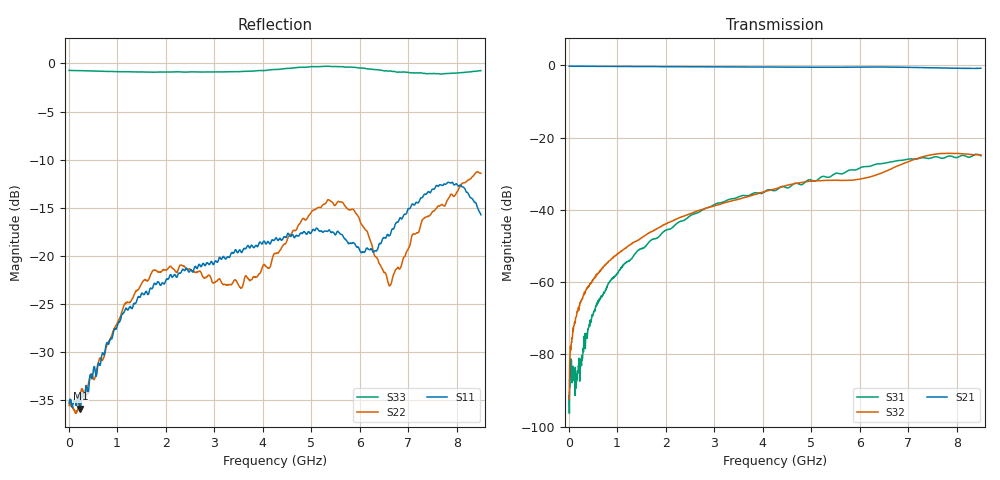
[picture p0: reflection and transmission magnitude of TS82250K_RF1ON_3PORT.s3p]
!Created with skrf (http://scikit-rf.org).
# GHz S RI R 50.0
!freq ReS11 ImS11 ReS12 ImS12 ReS13 ImS13
! ReS21 ImS21 ReS22 ImS22 ReS23 ImS23
! ReS31 ImS31 ReS32 ImS32 ReS33 ImS33
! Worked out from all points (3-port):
!   1601 points, 10 MHz to 8.5 GHz, reference 50 ohm
!   strongest paths, dB at 10 MHz, 2.132 GHz, 4.255 GHz, 6.378 GHz, 8.5 GHz:
!     S21: -0.2, -0.3, -0.4, -0.4, -0.8
!     S32: -92.4, -43.1, -34.2, -30.2, -24.7
!     S31: -91.5, -45.0, -34.6, -27.2, -25.0
!   lowest |S11| = -35.9 dB at 243.5 MHz (marker M1), VSWR 1.03, Z = 51.5 + j0.62 ohm
!   |S11| at or under -10 dB: start of sweep to end of sweep
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0.01  0.0172 -0.000587  0.9786 -0.0047  2.16e-05 3.25e-05
      0.9785 -0.00476  0.0166 0.00172  1.27e-05 5.26e-05
      1.5e-05 2.18e-05  1.21e-05 2.08e-05  -0.9197 0.00518
0.243475  0.0149 0.00601  0.9728 -0.069  -3.85e-05 6.52e-05
          0.9729 -0.069  0.018 0.00689  3.4e-05 0.00052
          -3.3e-05 6.45e-05  3.84e-05 0.000518  -0.9102 0.1129
0.6096063  0.0202 0.0184  0.9585 -0.1687  -0.000423 0.000312
           0.9585 -0.1686  0.0205 0.0187  -8.48e-05 0.00134
           -0.00048 0.000288  -8.95e-05 0.00134  -0.8707 0.2708
1.437381  0.0408 0.046  0.8882 -0.3828  -0.00235 0.0015
          0.8878 -0.3825  0.0406 0.0532  -0.000381 0.00384
          -0.00234 0.00149  -0.000397 0.00382  -0.6938 0.5779
3.034562  0.0919 0.0208  0.6324 -0.7172  -0.00679 0.0101
          0.6328 -0.7165  0.0504 0.0533  0.00266 0.0112
          -0.00677 0.0101  0.00277 0.0112  -0.1917 0.8826
4.255  0.1219 0.00724  0.3482 -0.8852  -0.00382 0.0181
       0.3479 -0.8847  0.0704 0.0754  0.0102 0.0167
       -0.0037 0.0182  0.0102 0.0167  0.2766 0.8865
5.602787  0.109 -0.0707  0.00603 -0.9458  0.000181 0.0317
          0.00608 -0.9457  0.1732 0.0797  0.022 0.0133
          0.000688 0.0317  0.022 0.0133  0.5265 0.8064
6.626894  -0.0509 -0.1174  -0.2788 -0.9094  0.0137 0.044
          -0.2793 -0.9087  0.0417 0.0563  0.0301 0.0205
          0.0145 0.0437  0.03 0.0204  0.6821 0.6078
7.831412  -0.1117 -0.2139  -0.5813 -0.7119  0.0408 0.0378
          -0.5812 -0.7128  0.1176 0.1604  0.0606 -0.00524
          0.0416 0.0368  0.0608 -0.00518  0.8538 0.2401
8.5  -0.0747 -0.1455  -0.7132 -0.5751  0.0509 0.0239
     -0.7128 -0.5744  0.2308 0.1367  0.0525 -0.0242
     0.0508 0.0239  0.0525 -0.0243  0.9138 0.0753
